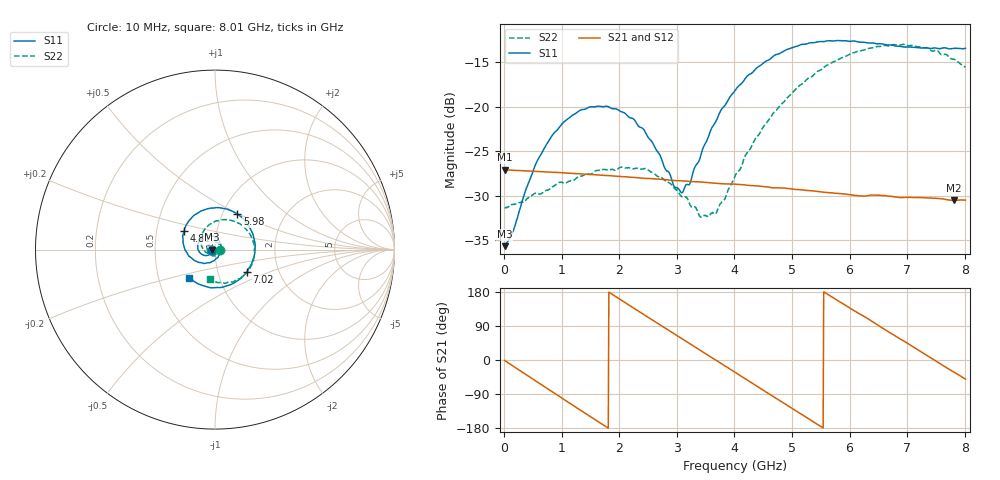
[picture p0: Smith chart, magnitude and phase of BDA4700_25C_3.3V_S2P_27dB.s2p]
!Agilent Technologies,E5071B,MY42404982,A.09.10
!Date: Mon Oct 20 18:14:25 2025
!Data & Calibration Information:
!Freq	S11:SOLT2(ON)	S21:SOLT2(ON)	S12:SOLT2(ON)	S22:SOLT2(ON)
# Hz S RI R 50
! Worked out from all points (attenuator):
!   801 points, 10 MHz to 8.01 GHz, reference 50 ohm
!   highest |S21| = -27.06 dB at 10 MHz (marker M1); lowest = -30.5 dB at 7.81 GHz (marker M2)
!   lowest |S11| = -35.6 dB at 10 MHz (marker M3), VSWR 1.03, Z = 48.4 - j0.101 ohm
!   |S11| at or under -10 dB: start of sweep to end of sweep
!   |S22| runs from -32.4 to -13.0 dB; largest |S21 - S12| = 0.00053
!   S11 on the Smith chart (normalised r, x): 10 MHz: 0.97, -0.00; 4.81 GHz: 0.69, +0.15; 5.98 GHz: 1.18, +0.49; 7.02 GHz: 1.37, -0.36; 8.01 GHz: 0.72, -0.24
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1e7  -0.0165 -0.00104  0.0443 -0.000968  0.0443 -0.000976  0.0272 -0.000782
1.5e8  -0.0175 -0.00944  0.0425 -0.0117  0.0424 -0.0117  0.0273 -0.00734
4e8  -0.026 -0.0243  0.0332 -0.0283  0.0332 -0.0283  0.0215 -0.0217
7e8  -0.0482 -0.0331  0.0145 -0.0407  0.0145 -0.0406  0.00615 -0.033
1.02e9  -0.0774 -0.0239  -0.00892 -0.0416  -0.00895 -0.0417  -0.0159 -0.034
1.35e9  -0.0962 0.00551  -0.0295 -0.0298  -0.0295 -0.0299  -0.0365 -0.0182
2.08e9  -0.0521 0.0768  -0.0363 0.018  -0.0363 0.018  -0.0302 0.0339
2.68e9  0.022 0.0506  -0.00368 0.0391  -0.00376 0.039  0.013 0.0384
2.96e9  0.0337 0.0111  0.0141 0.0359  0.0141 0.0358  0.0261 0.0231
3.1e9  0.0313 -0.0106  0.0221 0.0314  0.0219 0.0315  0.0289 0.0117
3.23e9  0.0238 -0.0287  0.028 0.0258  0.0281 0.0257  0.028 0.00267
3.54e9  -0.0139 -0.0653  0.0366 0.00826  0.0367 0.00825  0.0142 -0.0197
3.69e9  -0.0406 -0.0737  0.0372 -0.00105  0.0373 -0.00119  0.00161 -0.0254
4.01e9  -0.1044 -0.0652  0.0311 -0.0197  0.0311 -0.0196  -0.0312 -0.0262
4.81e9  -0.1724 0.1032  -0.0116 -0.033  -0.0114 -0.0331  -0.0777 0.0677
5.35e9  -0.0707 0.2175  -0.032 -0.0109  -0.0319 -0.011  -0.0157 0.147
5.98e9  0.125 0.1969  -0.0244 0.021  -0.0245 0.0209  0.1262 0.1491
6.68e9  0.2215 -0.0133  0.00877 0.0302  0.00881 0.0303  0.2195 0.000309
7.02e9  0.1763 -0.1252  0.0228 0.021  0.0229 0.0209  0.2005 -0.0909
7.45e9  0.0467 -0.2083  0.0306 0.000954  0.0307 0.000938  0.1132 -0.171
7.81e9  -0.0824 -0.1959  0.0254 -0.0156  0.0254 -0.0156  0.0173 -0.1842
8.01e9  -0.1425 -0.1577  0.0191 -0.023  0.0192 -0.023  -0.0301 -0.1637
